[IBIS Ver]   3.2
[File Name]   sprm142.ibs
[File Rev]   0.6
[Date]   July 31, 2008
[Source]   IBIS Model Generated from PACED 4.51D
[Disclaimer]   Please be aware that in the absence of a written agreement
|   Texas Instruments(TI) assumes no liability for:
|   (1) The accuracy of the IBIS models provided to your company
|   (2) The proper functioning of these Models in your design
|   or for any resulting applications; or
|   (3)Infringement of patents, copyrights or intellectual
|   property rights resulting from your use of these models.
|   TI provides IBIS Models as a service to our customers and
|   therefore reserves the right to limit distribution of the
|   Models.
[Copyright]   Property of Texas Instruments Incorporated.
|   Unauthorized reproduction and/or distribution is strictly.
|   prohibited.
|   This product is protected under copyright law and trade
|   secret law as an unpublished work.
|   Created 2002,(C) Copyright 2002,
|   Texas Instruments Incorporated., All Rights Reserved.
|   These commodities are under the U.S.
|   Government distribution license control. As such,they are
|   not to be re-exported without the prior approval of the U.S.
|   Department of Commerce.
[Notes]   Revision History
|   0.4  Updated CLKOUT3 buffer to reflect silicon revision 2.0
|   for C6713B GDP device.
|   0.5  Added OUK831PE1001 buffer definition.
|   0.6  Fixed swapped min/max values for UOS335PE1001 C_comp
[Component]   c6713B_GDP
[Manufacturer]   Texas Instruments
[Package]
| Variable   Typ   Min   Max
R_pkg   0.15798   0.1249   0.19129
L_pkg   4.816e-09   3.586e-09   6.029e-09
C_pkg   1.362e-12   8.298e-13   1.789e-12
[Pin] signal_name   model_name   R_pin   L_pin   C_pin
A3   CLKIN   IDH091PE1001   0.18019   5.664E-09   1.7625E-12
Y12   CLKOUT2/GP2   IDH091UOS335PE1001  0.16709   5.124E-09   1.4203E-12
D10   CLKOUT3   OUK831PE1001   0.12485   3.586E-09   9.165E-13
C4   CLKMODE0   IDH091PS1001   0.15399   4.656E-09   1.3457E-12
B7   TMS   IDH091PS1001   0.15672   4.757E-09   1.3298E-12
A8   TDO   OUK831PS1001   0.16876   5.201E-09   1.4526E-12
A7   TDI   IDH091PS1001   0.17187   5.326E-09   1.4901E-12
A6   TCK   IDH091PS1001   0.17452   5.436E-09   1.563E-12
B6   TRSTz   IDH091PE1001   0.15745   4.805E-09   1.3514E-12
B12   EMU5   IDH091OUK831PS1001  0.1503   4.526E-09   1.2197E-12
C11   EMU4   IDH091OUK831PS1001  0.13457   3.948E-09   1.034E-12
B10   EMU3   IDH091OUK831PS1001  0.14073   4.347E-09   1.3521E-12
D3   EMU2   IDH091OUK831PS1001  0.15496   4.735E-09   1.2636E-12
B9   EMU1   IDH091OUK831PS1001  0.15386   4.643E-09   1.2548E-12
D9   EMU0   IDH091OUK831PS1001  0.12688   3.663E-09   9.161E-13
A13   RESETz   IDG091PS1001   0.1637   5.019E-09   1.3754E-12
C13   NMI   IDH091PE1001   0.139   4.115E-09   1.1233E-12
E3   GP7   IDH091OUK831PS1001  0.14773   4.469E-09   1.2867E-12
D2   GP6   IDH091OUK831PS1001  0.16895   5.218E-09   1.4683E-12
C1   GP5/AMUTEIN0   IDH091OUK831PS1001  0.17903   5.639E-09   1.7233E-12
C2   GP4/AMUTEIN1   IDH091OUK831PS1001  0.15766   4.795E-09   1.383E-12
J20   HINTz/GP1   IDH091OUK831PS1001  0.16593   5.115E-09   1.3986E-12
G19   HCNTRL1/AXR1_1 IDH091OUK831PS1001  0.15904   4.822E-09   1.3741E-12
G18   HCNTRL0/AXR1_3 IDH091OUK831PS1001  0.14411   4.29E-09   1.1745E-12
H20   HHWIL/AFSR1   IDH091OUK831PS1001  0.16817   5.178E-09   1.4698E-12
G20   HRW/AXR1_0   IDH091OUK831PS1001  0.17246   5.313E-09   1.5186E-12
B14   HD15/GP15   IDH091OUK831PS1001  0.15614   4.74E-09   1.3503E-12
C14   HD14/GP14   IDH091OUK831PS1001  0.14248   4.263E-09   1.1586E-12
A15   HD13/GP13   IDH091OUK831PS1001  0.16971   5.261E-09   1.4942E-12
C15   HD12/GP12   IDH091OUK831PS1001  0.14322   4.168E-09   8.996E-13
A16   HD11/GP11   IDH091OUK831PS1001  0.17527   5.47E-09   1.6047E-12
B16   HD10/GP10   IDH091OUK831PS1001  0.16097   4.936E-09   1.4722E-12
C16   HD9/GP9   IDH091OUK831PS1001  0.14887   4.532E-09   1.2756E-12
B17   HD8/GP8   IDH091OUK831PS1001  0.16682   5.182E-09   1.4812E-12
A18   HD7/GP3   IDH091OUK831PS1001  0.18133   5.701E-09   1.7498E-12
C17   HD6/AHCLKR1   IDH091OUK831PS1001  0.14096   4.256E-09   1.1341E-12
B18   HD5/AHCLKX1   IDH091OUK831PS1001  0.17123   5.328E-09   1.5329E-12
C19   HD4/GP0   IDH091OUK831PE1001  0.15648   4.727E-09   1.4246E-12
C20   HD3/AMUTE1   IDH091OUK831PS1001  0.19129   6.029E-09   1.7775E-12
D18   HD2/AFSX1   IDH091OUK831PS1001  0.15791   4.798E-09   1.404E-12
D20   HD1/AXR1_7   IDH091OUK831PS1001  0.18476   5.778E-09   1.7108E-12
E20   HD0/AXR1_4   IDH091OUK831PS1001  0.17664   5.467E-09   1.5785E-12
E18   HASz/ACLKX1   IDH091OUK831PS1001  0.15619   4.704E-09   1.3866E-12
F20   HCSz/AXR1_2   IDH091OUK831PS1001  0.17499   5.405E-09   1.5549E-12
E19   HDS1z/AXR1_6   IDH091OUK831PS1001  0.16748   5.153E-09   1.4861E-12
F18   HDS2z/AXR1_5   IDH091OUK831PS1001  0.14984   4.514E-09   1.241E-12
H19   HRDYz/ACLKR1   IDH091OUK831PE1001  0.15532   4.706E-09   1.3004E-12
V6   CE3z   IDH091OUK831PS1001  0.14621   4.39E-09   1.2151E-12
W6   CE2z   IDH091OUK831PS1001  0.16098   4.921E-09   1.4132E-12
W18   CE1z   IDH091OUK831PS1001  0.17556   5.446E-09   1.6489E-12
V17   CE0z   IDH091OUK831PS1001  0.15744   4.8E-09   1.3798E-12
V5   BE3z   IDH091OUK831PS1001  0.151   4.541E-09   1.3313E-12
Y4   BE2z   IDH091OUK831PS1001  0.18214   5.702E-09   1.7154E-12
U19   BE1z   IDH091OUK831PS1001  0.16093   4.997E-09   1.4815E-12
V20   BE0z   IDH091OUK831PS1001  0.17611   5.497E-09   1.6313E-12
J18   HOLDAz   IDH091OUK831PS1001  0.14188   4.206E-09   1.1141E-12
J17   HOLDz   IDH091OUK831PS1001  0.13083   3.807E-09   9.644E-13
J19   BUSREQ   IDH091OUK831PS1001  0.14582   4.359E-09   1.1679E-12
Y11   ECLKIN   IDH091PE1001   0.16208   0.000000005   1.4122E-12
Y10   ECLKOUT   UOS335PE1001   0.16106   4.931E-09   1.345E-12
V11   SDCASz   IDH091OUK831PS1001  0.1364   4.059E-09   1.03E-12
W10   SDRASz   IDH091OUK831PS1001  0.1486   4.45E-09   1.1911E-12
V12   SDWEz   IDH091OUK831PS1001  0.14012   4.139E-09   1.0969E-12
Y5   ARDY   IDH091OUK831PS1001  0.17592   5.451E-09   1.6354E-12
U18   EA21   IDH091OUK831PS1001  0.13802   4.156E-09   1.129E-12
Y18   EA20   IDH091OUK831PS1001  0.18588   5.849E-09   1.7404E-12
W17   EA19   IDH091OUK831PS1001  0.16927   5.225E-09   1.5492E-12
Y16   EA18   IDH091OUK831PS1001  0.17911   5.584E-09   1.6036E-12
V16   EA17   IDH091OUK831PS1001  0.15217   4.613E-09   1.3114E-12
Y15   EA16   IDH091OUK831PS1001  0.17574   5.447E-09   1.5678E-12
W15   EA15   IDH091OUK831PS1001  0.16072   4.894E-09   1.4026E-12
Y14   EA14   IDH091OUK831PS1001  0.1722   5.313E-09   1.5193E-12
W14   EA13   IDH091OUK831PS1001  0.15855   4.806E-09   1.3767E-12
V14   EA12   IDH091OUK831PS1001  0.14298   4.247E-09   1.1833E-12
W13   EA11   IDH091OUK831PS1001  0.15509   4.674E-09   1.3133E-12
V10   EA10   IDH091OUK831PS1001  0.1353   3.969E-09   1.0187E-12
Y9   EA9   IDH091OUK831PS1001  0.1646   5.033E-09   1.4055E-12
V9   EA8   IDH091OUK831PS1001  0.13792   4.071E-09   1.0499E-12
Y8   EA7   IDH091OUK831PS1001  0.16615   5.125E-09   1.4253E-12
W8   EA6   IDH091OUK831PS1001  0.1525   4.599E-09   1.2789E-12
V8   EA5   IDH091OUK831PS1001  0.14065   4.164E-09   1.1235E-12
W7   EA4   IDH091OUK831PS1001  0.15712   4.787E-09   1.3445E-12
V7   EA3   IDH091OUK831PS1001  0.1433   4.261E-09   1.1748E-12
Y6   EA2   IDH091OUK831PS1001  0.17352   5.39E-09   1.5923E-12
N3   ED31   IDH091OUK831PS1001  0.14113   4.183E-09   1.148E-12
P3   ED30   IDH091OUK831PS1001  0.14174   4.207E-09   1.1817E-12
P2   ED29   IDH091OUK831PS1001  0.15844   4.811E-09   1.3892E-12
P1   ED28   IDH091OUK831PS1001  0.17146   5.291E-09   1.5266E-12
R2   ED27   IDH091OUK831PS1001  0.15673   4.761E-09   1.376E-12
R3   ED26   IDH091OUK831PS1001  0.14413   4.353E-09   1.2565E-12
T2   ED25   IDH091OUK831PS1001  0.16136   4.962E-09   1.5047E-12
T1   ED24   IDH091OUK831PS1001  0.16908   5.22E-09   1.4934E-12
U3   ED23   IDH091OUK831PS1001  0.1553   4.77E-09   1.3843E-12
U1   ED22   IDH091OUK831PS1001  0.17507   5.452E-09   1.6882E-12
U2   ED21   IDH091OUK831PS1001  0.16682   5.182E-09   1.5635E-12
V1   ED20   IDH091OUK831PS1001  0.18101   5.699E-09   1.7157E-12
V2   ED19   IDH091OUK831PS1001  0.17526   5.479E-09   1.6486E-12
Y3   ED18   IDH091OUK831PS1001  0.18871   5.998E-09   1.7365E-12
W4   ED17   IDH091OUK831PS1001  0.16804   5.371E-09   1.7892E-12
V4   ED16   IDH091OUK831PS1001  0.13857   4.01E-09   8.298E-13
T19   ED15   IDH091OUK831PS1001  0.16189   4.967E-09   1.4499E-12
T20   ED14   IDH091OUK831PS1001  0.17215   5.387E-09   1.5831E-12
T18   ED13   IDH091OUK831PS1001  0.15033   4.53E-09   1.3312E-12
R20   ED12   IDH091OUK831PS1001  0.17084   5.33E-09   1.5388E-12
R19   ED11   IDH091OUK831PS1001  0.15882   4.87E-09   1.3707E-12
P20   ED10   IDH091OUK831PS1001  0.16585   5.138E-09   1.4498E-12
P18   ED9   IDH091OUK831PS1001  0.14348   4.278E-09   1.1512E-12
N20   ED8   IDH091OUK831PS1001  0.16474   5.075E-09   1.4344E-12
N19   ED7   IDH091OUK831PS1001  0.15249   4.606E-09   1.2735E-12
N18   ED6   IDH091OUK831PS1001  0.1392   4.109E-09   1.0975E-12
M20   ED5   IDH091OUK831PS1001  0.16351   4.995E-09   1.4105E-12
M19   ED4   IDH091OUK831PS1001  0.15158   4.535E-09   1.2513E-12
L19   ED3   IDH091OUK831PS1001  0.15121   4.529E-09   1.2368E-12
L18   ED2   IDH091OUK831PS1001  0.13524   3.962E-09   1.023E-12
K19   ED1   IDH091OUK831PS1001  0.14992   4.542E-09   1.2211E-12
K18   ED0   IDH091OUK831PS1001  0.13736   4.069E-09   1.0426E-12
F1   TOUT1/AXR0_4   IDH091OUK831PE1001  0.17453   5.437E-09   1.5615E-12
F2   TINP1/AHCLKX0  IDH091OUK831PE1001  0.15861   4.866E-09   1.3778E-12
G1   TOUT0/AXR0_2   IDH091OUK831PE1001  0.16999   5.241E-09   1.5004E-12
G2   TINP0/AXR0_3   IDH091OUK831PE1001  0.15603   4.739E-09   1.3418E-12
E1   CLKS1/SCL1   IDG091UOS205   0.17483   5.458E-09   1.617E-12
M1   CLKR1/AXR0_6   IDH091OUK831PE1001  0.16737   5.138E-09   1.4594E-12
L3   CLKX1/AMUTE0   IDH091OUK831PE1001  0.13844   4.083E-09   1.0869E-12
M2   DR1/SDA1   IDG091UOS205   0.15325   4.608E-09   1.3011E-12
L2   DX1/AXR0_5   IDH091OUK831PS1001  0.15147   4.517E-09   1.3075E-12
M3   FSR1/AXR0_7   IDH091OUK831PE1001  0.13992   4.134E-09   1.1163E-12
L1   FSX1   IDH091OUK831PE1001  0.16353   4.946E-09   1.4648E-12
K3   CLKS0/AHCLKR0  IDH091OUK831PE1001  0.13597   4.005E-09   1.0142E-12
H3   CLKR0/ACLKR0   IDH091OUK831PE1001  0.13887   4.103E-09   1.1188E-12
G3   CLKX0/ACLKX0   IDH091OUK831PE1001  0.14227   4.232E-09   1.1737E-12
J1   DR0/AXR0_0   IDH091OUK831PS1001  0.16689   5.141E-09   1.3597E-12
H2   DX0/AXR0_1   IDH091OUK831PS1001  0.15223   4.578E-09   1.31E-12
J3   FSR0/AFSR0   IDH091OUK831PE1001  0.13605   4.002E-09   1.0327E-12
H1   FSX0/AFSX0   IDH091OUK831PE1001  0.16688   5.126E-09   1.4562E-12
N1   SCL0   IDG091UOS205   0.16821   5.18E-09   1.4761E-12
N2   SDA0   IDG091UOS205   0.15572   4.719E-09   1.3287E-12
| End of package information
| Component   IDG091PS1001
[Component]   IDG091PS1001
[Manufacturer]   Texas Instruments
[Package]
|   typ   min   max
R_pkg   0   0   0
L_pkg   0   0   0
C_pkg   0   0   0
[Pin]   signal_name   model_name   R_pin   L_pin   C_pin
   1   A   IDG091PS1001   0   0   0
| Component   IDG091UOS205
[Component]   IDG091UOS205
[Manufacturer]   Texas Instruments
[Package]
|   typ   min   max
R_pkg   0   0   0
L_pkg   0   0   0
C_pkg   0   0   0
[Pin]   signal_name   model_name   R_pin   L_pin   C_pin
   1   Y   IDG091UOS205   0   0   0
| Component   IDH091OUK831PE1001
[Component]   IDH091OUK831PE1001
[Manufacturer]   Texas Instruments
[Package]
|   typ   min   max
R_pkg   0   0   0
L_pkg   0   0   0
C_pkg   0   0   0
[Pin]   signal_name   model_name   R_pin   L_pin   C_pin
   1   Y  IDH091OUK831PE1001   0   0   0
| Component   IDH091OUK831PS1001
[Component]   IDH091OUK831PS1001
[Manufacturer]   Texas Instruments
[Package]
|   typ   min   max
R_pkg   0   0   0
L_pkg   0   0   0
C_pkg   0   0   0
[Pin]   signal_name   model_name   R_pin   L_pin   C_pin
   1   Y  IDH091OUK831PS1001   0   0   0
| Component   IDH091PE1001
[Component]   IDH091PE1001
[Manufacturer]   Texas Instruments
[Package]
|   typ   min   max
R_pkg   0   0   0
L_pkg   0   0   0
C_pkg   0   0   0
[Pin]   signal_name   model_name   R_pin   L_pin   C_pin
   1   A   IDH091PE1001   0   0   0
| Component   IDH091PS1001
[Component]   IDH091PS1001
[Manufacturer]   Texas Instruments
[Package]
|   typ   min   max
R_pkg   0   0   0
L_pkg   0   0   0
C_pkg   0   0   0
[Pin]   signal_name   model_name   R_pin   L_pin   C_pin
   1   A   IDH091PS1001   0   0   0
| Component   IDH091UOS335PE1001
[Component]   IDH091UOS335PE1001
[Manufacturer]   Texas Instruments
[Package]
|   typ   min   max
R_pkg   0   0   0
L_pkg   0   0   0
C_pkg   0   0   0
[Pin]   signal_name   model_name   R_pin   L_pin   C_pin
   1   Y  IDH091UOS335PE1001   0   0   0
| Component   OUK831PS1001
[Component]   OUK831PS1001
[Manufacturer]   Texas Instruments
[Package]
|   typ   min   max
R_pkg   0   0   0
L_pkg   0   0   0
C_pkg   0   0   0
[Pin]   signal_name   model_name   R_pin   L_pin   C_pin
   1   Y   OUK831PS1001   0   0   0
| Component   UOS335PE1001
[Component]   UOS335PE1001
[Manufacturer]   Texas Instruments
[Package]
|   typ   min   max
R_pkg   0   0   0
L_pkg   0   0   0
C_pkg   0   0   0
[Pin]   signal_name   model_name   R_pin   L_pin   C_pin
   1   Y   UOS335PE1001   0   0   0
| Component   OUK831PE1001
[Component]   OUK831PE1001
[Manufacturer]   Texas Instruments
[Package]
|   typ   min   max
R_pkg   0   0   0
L_pkg   0   0   0
C_pkg   0   0   0
[Pin]   signal_name   model_name   R_pin   L_pin   C_pin
   1   Y   OUK831PE1001   0   0   0
| Models and submodels in the file (10): IDG091PS1001 (Input), IDG091UOS205 (I/O_open_drain), IDH091OUK831PE1001 (I/O), IDH091OUK831PS1001 (I/O), IDH091PE1001 (Input), IDH091PS1001 (Input), IDH091UOS335PE1001 (I/O), OUK831PS1001 (3-state), UOS335PE1001 (3-state), OUK831PE1001 (3-state)
